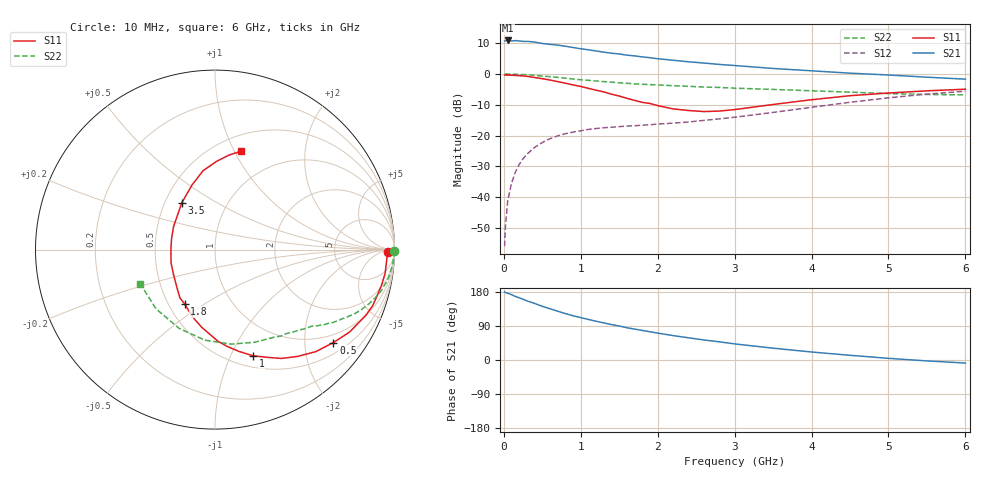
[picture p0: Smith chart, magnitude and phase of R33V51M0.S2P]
! SIEMENS Small Signal Semiconductors
! BFR181
! Si NPN RF Bipolar Junction Transistor in SOT23
! VCE = 3.5 V  IC = 1 mA
! Common Emitter S-Parameters:  May  1996
# GHz  S  MA  R  50
!  f  S11  S21  S12  S22
! GHz  MAG  ANG  MAG  ANG  MAG  ANG  MAG  ANG
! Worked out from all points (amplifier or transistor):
!   36 points, 10 MHz to 6 GHz, reference 50 ohm
!   highest |S21| = 10.9 dB at 50 MHz (marker M1)
!   |S21| within 3 dB of that: start of sweep to 1.09 GHz
!   unconditionally stable (mu >= 1): 2.022 GHz to 3.666 GHz
!   at 250 MHz: K = 0.15, MSG = 19.1 dB, |S12| = -27.5 dB
!   at 1.4 GHz: K = 0.77, MSG = 12.0 dB, |S12| = -17.3 dB
!   at 6 GHz: K = 0.87, MSG = 2.0 dB, |S12| = -5.6 dB
!   lowest NFmin = 1.30 dB at 450 MHz
!   S11 on the Smith chart (normalised r, x): 10 MHz: 46, -17; 500 MHz: 0.77, -2.70; 1 GHz: 0.62, -1.22; 1.8 GHz: 0.60, -0.41; 3.5 GHz: 0.61, +0.36; 6 GHz: 0.66, +1.06
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0.01  0.9622 -0.8  3.429 179.5  0.0016 93.1  0.9992 -0.4
0.02  0.9605 -1.6  3.464 178.3  0.0033 86.3  0.9983 -0.8
0.05  0.9581 -4.0  3.509 176.2  0.0087 86.7  0.998 -1.9
0.1  0.9571 -7.9  3.448 172.5  0.0169 84.6  0.9948 -3.7
0.15  0.9494 -11.8  3.487 167.7  0.0255 81.8  0.9901 -5.6
0.2  0.9401 -15.6  3.442 164.1  0.034 79.9  0.9846 -7.4
0.3  0.9166 -23.6  3.387 156.0  0.0499 75.1  0.971 -10.9
0.4  0.8793 -31.5  3.309 149.3  0.0643 70.2  0.9514 -14.3
0.5  0.8389 -38.1  3.131 141.6  0.0771 65.7  0.9276 -17.3
0.7  0.753 -52.2  2.949 128.8  0.099 58.7  0.8797 -22.5
0.8  0.7104 -58.6  2.824 122.5  0.1076 55.4  0.8555 -24.7
1  0.6282 -70.3  2.572 111.8  0.1198 50.8  0.8074 -28.5
1.1  0.5851 -76.4  2.475 107.0  0.1261 48.9  0.7893 -30.2
1.4  0.4695 -94.0  2.174 93.4  0.1368 45.0  0.7371 -34.6
1.8  0.3466 -119.3  1.897 78.0  0.1477 44.2  0.682 -39.1
2.2  0.2714 -148.0  1.674 64.4  0.1593 45.6  0.6461 -44.1
2.6  0.2456 178.9  1.508 52.9  0.1766 48.3  0.6145 -49.5
3  0.2644 150.7  1.375 42.5  0.1989 50.5  0.5891 -55.9
3.5  0.3203 125.2  1.231 31.2  0.238 51.7  0.5624 -66.5
4.5  0.4446 98.6  1.033 12.4  0.3475 47.4  0.5077 -96.5
5.5  0.5334 81.4  0.888 -2.4  0.4711 34.9  0.4657 -134.7
6  0.5668 75.1  0.826 -8.0  0.5261 27.0  0.4582 -155.1
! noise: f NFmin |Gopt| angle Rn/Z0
0.45  1.3  0.7  18  0.5
0.9  1.4  0.6  39  0.52
1.8  1.85  0.4  81  0.47
